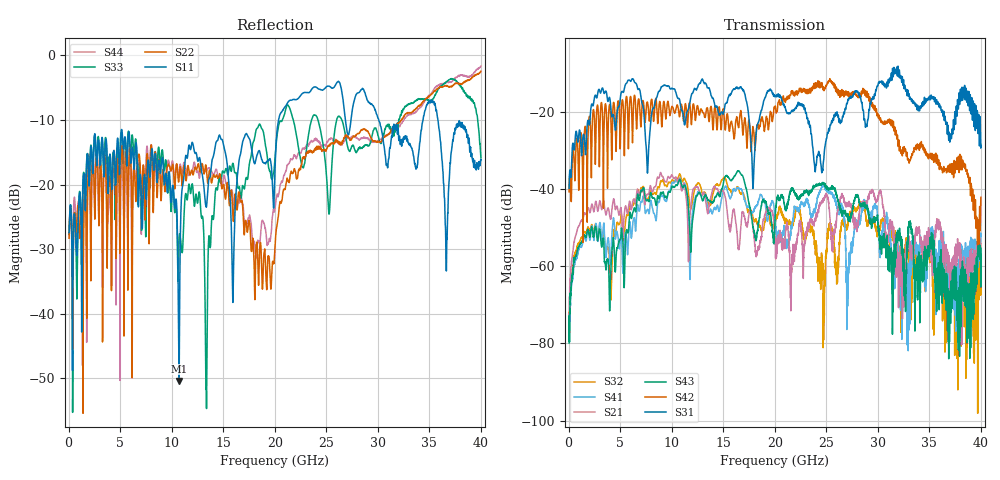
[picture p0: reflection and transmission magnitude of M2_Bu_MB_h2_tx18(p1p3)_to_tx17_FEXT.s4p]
! S11 = S11
! S12 = S12
! S13 = S13
! S14 = S14
! S21 = S21
! S22 = S22
! S23 = S23
! S24 = S24
! S31 = S31
! S32 = S32
! S33 = S33
! S34 = S34
! S41 = S41
! S42 = S42
! S43 = S43
! S44 = S44
! FILE: \\englab.brocade.com\shares\Groups\SIT\Work\Shaohua\IEEE_channels\M2_Bu_MB_h2_tx18(p1p3)_to_tx17_FEXT.s4p
!$DUT_CFG_DESC: Default 4-Port Configuration
!$NUMBER_PORTS: 4
!$DIFF_PORT_MAP: 1|2P|2|2P|0|UC|0|UC|
!$PORT_MAP: PNA 1|1|<<<<<<|TS 2|2|>>>>>>|PNA 2|3|<<<<<<|TS 4|4|>>>>>>|
# MHz S RI R 50.00
! FREQ  S11  S12  S13  S14
!  S21  S22  S23  S24
!  S31  S32  S33  S34
!  S41  S42  S43  S44
!  REAL  IMAG  REAL  IMAG  REAL  IMAG  REAL  IMAG
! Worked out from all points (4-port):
!   3996 points, 50 MHz to 40 GHz, reference 50 ohm
!   strongest paths, dB at 50 MHz, 10.04 GHz, 20.03 GHz, 30.02 GHz, 40 GHz:
!     S31: -39.8, -13.9, -16.1, -13.0, -28.7
!     S42: -40.7, -18.6, -18.7, -20.9, -42.2
!     S43: -79.9, -39.4, -47.8, -49.1, -57.0
!     S21: -72.3, -36.4, -53.6, -42.4, -54.1
!     S41: -78.7, -38.3, -47.1, -49.2, -51.5
!     S32: -76.1, -37.7, -47.3, -50.6, -63.5
!   lowest |S11| = -50.4 dB at 10.72 GHz (marker M1), VSWR 1.01, Z = 49.8 + j0.193 ohm
!   |S11| at or under -10 dB: start of sweep to 20.36 GHz; 30.09 GHz to 34.39 GHz (4.3 GHz wide, 13.3 % of centre); 35.84 GHz to end of sweep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
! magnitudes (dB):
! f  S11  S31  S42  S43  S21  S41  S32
! 50 MHz  -27.4  -39.8  -40.7  -79.9  -72.3  -78.7  -76.1
! 10.72 GHz  -50.4  -16.6  -20.9  -37.7  -37.2  -37.5  -36.4
! 21.6 GHz  -6.9  -20.0  -14.7  -40.0  -63.0  -50.2  -49.6
! 24.73 GHz  -5.3  -32.9  -13.6  -38.5  -42.9  -39.2  -74.0
! 27.1 GHz  -12.2  -16.8  -15.9  -47.4  -44.3  -63.0  -48.9
! 28.67 GHz  -5.5  -22.2  -14.5  -43.5  -43.6  -42.7  -44.9
! 40 GHz  -16.2  -28.7  -42.2  -57.0  -54.1  -51.5  -63.5
